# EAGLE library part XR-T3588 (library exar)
V.35/BELL 306 DRIVER/RECEIVER
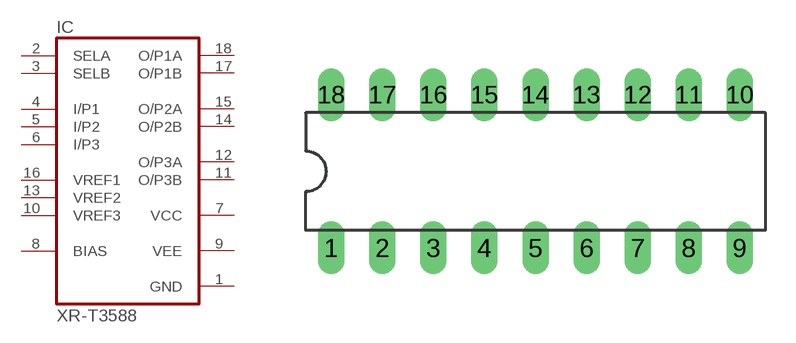
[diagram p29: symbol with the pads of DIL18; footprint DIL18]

Designator prefix IC

## XR-T3588 (OC_FARNELL: unknown; OC_NEWARK: unknown)  [DIL18]
1  GND  pwr
2  SELA  in
3  SELB  in
4  I/P1  in
5  I/P2  in
6  I/P3  in
7  VCC  pwr
8  BIAS  in
9  VEE  pwr
10  VREF3  in
11  O/P3B  out
12  O/P3A  out
13  VREF2  in
14  O/P2B  out
15  O/P2A  out
16  VREF1  in
17  O/P1B  out
18  O/P1A  out

## Footprint DIL18 (pad centres in mm)
Dual In Line Package
drill 0.813 long: 1 -10.16,-3.81; 2 -7.62,-3.81; 3 -5.08,-3.81; 4 -2.54,-3.81; 5 0,-3.81; 6 2.54,-3.81; 7 5.08,-3.81; 8 7.62,-3.81; 9 10.16,-3.81; 10 10.16,3.81; 11 7.62,3.81; 12 5.08,3.81; 13 2.54,3.81; 14 0,3.81; 15 -2.54,3.81; 16 -5.08,3.81; 17 -7.62,3.81; 18 -10.16,3.81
